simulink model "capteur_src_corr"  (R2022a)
settings: Solver=VariableStepAuto  StartTime=0.0  StopTime=10.0  RelTol=1e-3
libraries: simulink_extras x1, simulink x1

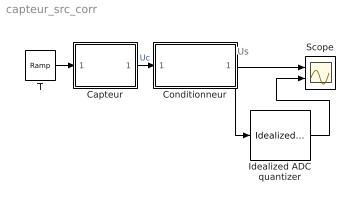
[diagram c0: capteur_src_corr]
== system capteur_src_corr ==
  note: Us
  Capteur : Subsystem
  Conditionneur : Subsystem
  Idealized ADC quantizer : simulink_extras/Additional Discrete/Idealized ADC quantizer  NumberOfConverterBits=4  Vmin=0  Vmax=5  OutputDataType=int16  OutputNegativeValues=off
  Scope : Scope  NumInputPorts=2
  T : simulink/Sources/Ramp  slope=13  start=0  InitialOutput=70
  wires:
  T/1 -> Capteur/1(T)
  Capteur/1(Uc) -> Conditionneur/1(Uc)  "Uc"
  Conditionneur/1(Us) -> Idealized ADC quantizer/1, Scope/1
  Idealized ADC quantizer/1 -> Scope/2

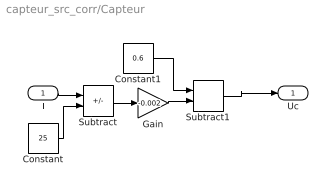
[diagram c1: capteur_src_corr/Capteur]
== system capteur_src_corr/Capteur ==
  T : Inport
  Constant : Constant  Value=25
  Constant1 : Constant  Value=0.6
  Gain : Gain  Gain=-0.002
  Subtract : Sum  Inputs=+-
  Subtract1 : Sum
  Uc : Outport
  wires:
  T/1 -> Subtract/1
  Constant/1 -> Subtract/2
  Subtract/1 -> Gain/1
  Gain/1 -> Subtract1/2
  Constant1/1 -> Subtract1/1
  Subtract1/1 -> Uc/1

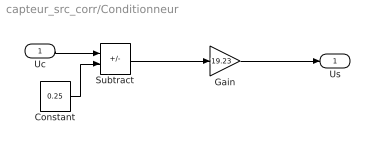
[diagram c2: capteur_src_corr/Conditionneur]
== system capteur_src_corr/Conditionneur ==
  Uc : Inport
  Constant : Constant  Value=0.25
  Gain : Gain  Gain=19.23
  Subtract : Sum  Inputs=+-
  Us : Outport
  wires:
  Uc/1 -> Subtract/1
  Constant/1 -> Subtract/2
  Subtract/1 -> Gain/1
  Gain/1 -> Us/1
